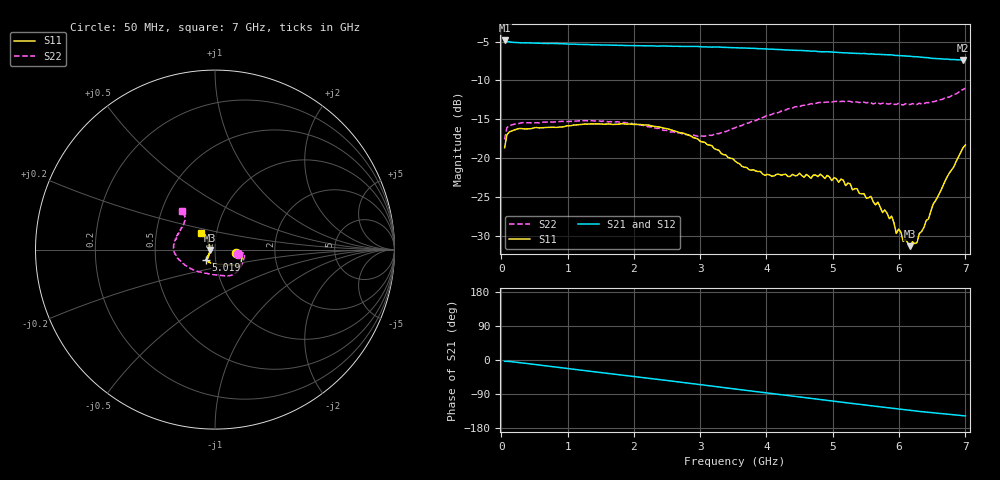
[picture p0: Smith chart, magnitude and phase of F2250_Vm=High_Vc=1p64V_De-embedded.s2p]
! Integrated Device Technology
! Corporate Headquarters
! 6024 Silver Creek Valley Road
! San Jose, CA 95138  USA
! Phone:  1-408-284-8200
! Toll Free:  1-800-223-1366
! Webpage:  http://www.idt.com/
! Timing and RF Division
! 515 Groton Road, Suite 102
! Westford, MA 01886-6024
! Device:  F2250
! Description: Voltage Variable RF Attenuator
! Frequency:  50.0 -  6000.00 MHz
! Package:  3x3 mm Thin QFN Plastic Package: 16 pin
! Ports:  2 RF, 3 DC
!  Pin  1  = GND
!  Pin  2  = NC
!  Pin  3  = RF1  = Port 1
!  Pin  4  = NC
!  Pin  5  = GND
!  Pin  6  = GND
!  Pin  7  = GND
!  Pin  8  = GND
!  Pin  9  = NC
!  Pin 10  = RF2  = Port 2
!  Pin 11  = NC
!  Pin 12  = GND
!  Pin 13  = GND
!  Pin 14  = VCNTRL
!  Pin 15  = VDD
!  Pin 16  = VMODE
! Vcntrl:  1.640 Volts
! Vmode:  +3.300 Volts
! Vdd:  +3.30  Volts
! Current:  1.327 mA
! Data:  The device was measured on a the F2250 evaluation board which has
!  individual transmission lines to the RF pins.  Data was collected
!  using a calibrated network analyzer.  The evaluation board was
!  de-embedded using a TRL calibration technique.
!  The reference plane is the edge of the package pin.
! Misc:  SN 10
!  Action Tracker AT0258
! Date Measured:  2014-11-26
! Date:  2015-10-15  MJV
! Note:
!  Integrated Device Technology supplies this data as a sample of measured
!  data at the package pin for this product.  Your particular data for this
!  product may vary.
!  Data was taken at 25 degrees C.
!  Integrated Device Technology reserves the right to change this data at anytime.
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# GHz S dB R 50
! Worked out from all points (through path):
!   201 points, 50 MHz to 7 GHz, reference 50 ohm
!   highest |S21| = -4.86 dB at 50 MHz (marker M1); lowest = -7.4 dB at 6.965 GHz (marker M2)
!   group delay of S21, straight-line fit = 59.2 ps
!   lowest |S11| = -31.3 dB at 6.166 GHz (marker M3), VSWR 1.06, Z = 47.4 - j0.158 ohm
!   |S11| at or under -10 dB: start of sweep to end of sweep
!   |S22| runs from -17.6 to -11.0 dB; largest |S21 - S12| = 0.0024
!   S11 on the Smith chart (normalised r, x): 50 MHz: 1.26, -0.05; 5.019 GHz: 0.90, -0.10; 7 GHz: 0.84, +0.16
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0.05  -18.67 -10.5  -4.86 -3.4  -4.88 -3.4  -17.61 -9.9
0.08475  -16.98 -6.1  -4.99 -3.4  -5.01 -3.4  -16.09 -6.7
0.2585  -16.21 -7.9  -5.14 -6.6  -5.16 -6.6  -15.55 -11.4
1.2315  -15.64 -27.2  -5.38 -27.5  -5.37 -27.5  -15.17 -43.3
2.37825  -15.99 -34.3  -5.58 -51.5  -5.58 -51.5  -16.17 -70.8
2.969  -17.56 -40.8  -5.63 -64.3  -5.67 -64.3  -17.19 -96.9
3.525  -20.37 -61.2  -5.79 -76.6  -5.80 -76.6  -16.11 -129.6
3.97675  -22.21 -89.6  -5.95 -86.5  -5.97 -86.5  -14.65 -151.3
4.7065  -22.19 -124.3  -6.24 -102.3  -6.24 -102.3  -13.03 -173.9
5.01925  -22.51 -131.0  -6.36 -109.0  -6.36 -109.0  -12.72 178.0
5.50575  -25.16 -134.5  -6.56 -119.2  -6.58 -119.2  -12.91 166.8
5.57525  -24.92 -135.1  -6.59 -120.5  -6.57 -120.7  -12.88 165.5
5.85325  -27.81 -143.6  -6.70 -126.4  -6.71 -126.5  -13.04 157.0
5.888  -27.47 -145.9  -6.71 -127.2  -6.74 -127.2  -12.93 157.1
5.9575  -29.69 -148.3  -6.78 -128.5  -6.78 -128.6  -13.09 154.2
5.99225  -29.14 -155.9  -6.79 -129.4  -6.80 -129.4  -12.96 153.8
6.06175  -30.70 -158.6  -6.83 -130.7  -6.85 -130.7  -13.16 151.0
6.166  -31.33 -176.5  -6.89 -132.8  -6.89 -132.9  -13.11 147.7
6.27025  -30.87 163.5  -6.96 -135.0  -6.96 -135.0  -13.09 144.3
6.5135  -25.92 134.2  -7.18 -139.5  -7.16 -139.7  -12.73 136.8
6.96525  -18.66 130.2  -7.38 -147.1  -7.38 -147.2  -11.17 131.4
7  -18.31 130.3  -7.36 -147.6  -7.38 -147.7  -11.01 130.6
